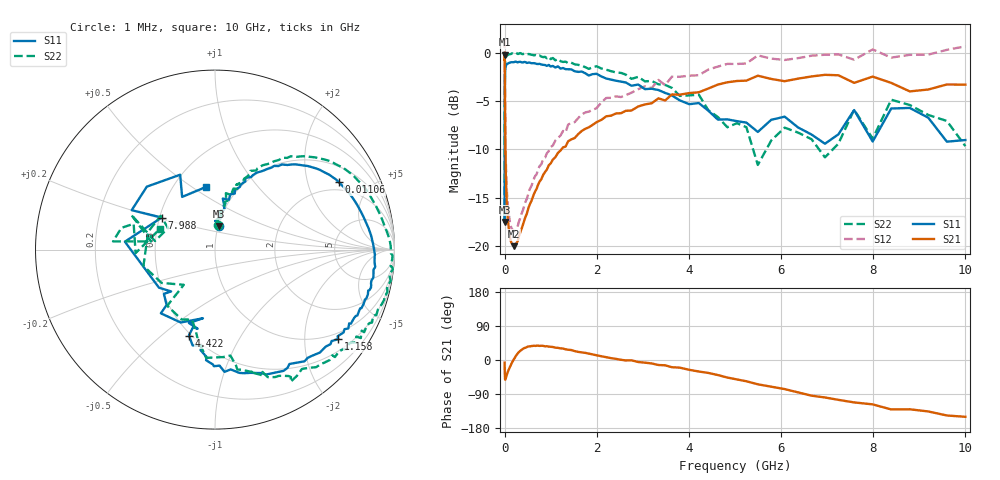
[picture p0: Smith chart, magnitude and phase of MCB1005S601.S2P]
!Agilent Technologies,E5071C,MY46111244,A.11.31
!Date: Tue May 07 14:56:41 2019
!Data & Calibration Information:
!Freq	S11:SOLT2(ON)	S21:SOLT2(ON)	S12:SOLT2(ON)	S22:SOLT2(ON)
# Hz S dB R 50
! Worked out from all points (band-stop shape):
!   201 points, 1 MHz to 10 GHz, reference 50 ohm
!   highest |S21| = -0.21 dB at 1.212 MHz (marker M1); lowest = -20.0 dB at 210.1 MHz (marker M2)
!   |S21| within 3 dB of the highest: start of sweep to 6.541 MHz; 4.718 GHz to 8.424 GHz (3.706 GHz wide, 56.4 % of centre)
!   lowest |S11| = -17.5 dB at 1 MHz (marker M3), VSWR 1.31, Z = 50.3 + j13.4 ohm
!   |S11| at or under -10 dB: start of sweep to 2.39 MHz
!   |S22| runs from -17.3 to 0.0 dB; largest |S21 - S12| = 0.49
!   S11 on the Smith chart (normalised r, x): 1 MHz: 1.01, +0.27; 11.06 MHz: 1.60, +3.15; 1.158 GHz: 0.81, -2.87; 4.422 GHz: 0.49, -0.62; 7.988 GHz: 0.51, +0.21; 10 GHz: 0.72, +0.57
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1000000  -17.53 81.1  -0.37 -7.1  1.07 -8.0  -17.33 82.1
1212171  -15.86 89.8  -0.21 -9.2  1.25 -10.1  -15.24 85.0
4810209  -5.13 55.5  -2.01 -33.6  -0.50 -34.4  -4.23 54.5
1.106086e7  -2.11 28.7  -6.50 -50.9  -4.96 -51.4  -1.16 27.9
2.206931e7  -1.51 14.4  -11.24 -49.8  -9.71 -50.3  -0.60 13.7
1.047129e8  -1.06 0.7  -18.67 -21.6  -17.16 -21.7  -0.18 0.1
2.101097e8  -0.99 -4.9  -20.03 3.7  -18.49 4.2  -0.15 -5.2
4.810209e8  -1.07 -15.0  -16.71 33.9  -15.15 35.0  -0.20 -15.2
1.158214e9  -1.43 -36.0  -10.38 32.0  -8.84 36.2  -0.65 -36.6
2.206931e9  -2.69 -69.7  -6.59 7.4  -4.69 13.2  -1.78 -59.8
4.421686e9  -6.02 -106.9  -3.72 -34.1  -1.76 -22.7  -5.97 -101.2
5.248075e9  -7.25 -109.6  -2.91 -56.1  -1.13 -43.2  -7.72 -130.4
5.495409e9  -8.21 -100.0  -2.40 -64.1  -0.30 -51.2  -11.63 -131.5
6.078392e9  -6.63 -130.4  -2.97 -76.8  -0.77 -62.7  -7.77 -167.2
6.661376e9  -8.48 -139.1  -2.47 -94.1  -0.33 -77.6  -8.96 148.2
7.24436e9  -8.46 -145.8  -2.35 -105.2  -0.19 -86.1  -9.43 171.8
7.585776e9  -5.95 175.0  -3.14 -111.9  -0.74 -96.2  -5.91 157.4
7.988146e9  -9.20 149.0  -2.49 -117.1  0.32 -100.0  -8.91 172.7
8.390517e9  -5.79 154.7  -3.14 -130.4  -0.52 -110.8  -4.88 175.4
9.195259e9  -6.74 115.0  -3.83 -135.8  -0.22 -118.8  -6.46 162.4
9.597629e9  -9.22 121.9  -3.30 -146.4  0.28 -126.5  -7.08 -177.5
1e10  -9.05 98.1  -3.32 -149.9  0.64 -130.3  -9.68 159.6
